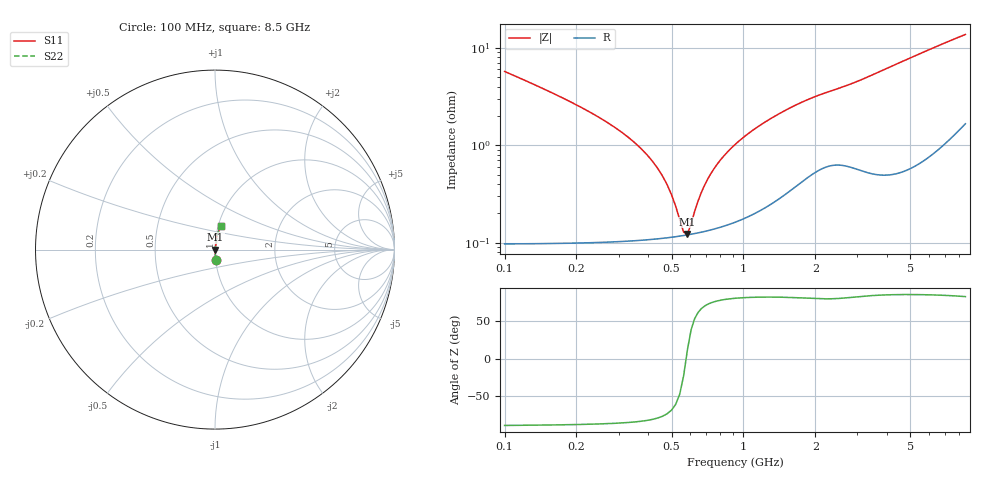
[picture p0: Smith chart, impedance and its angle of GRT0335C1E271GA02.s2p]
!Murata Part Number: GRT0335C1E271GA02
!These Parameters are Measured in Series Mode Connection
!Data Generated on Jun 19, 2026
!  o--ll--o
!Port1  Port2
!  o------o
!Operation Temp=25[degC], DC Bias Voltage=0[V]
!Freq. Start=100[MHz] Stop=9[GHz] 401[Steps]
# Hz S RI R 50
!Freq.(Hz) S11(Real) S11(Imag) S21(Real) S21(Imag) S12(Real) S12(Imag) S22(Real) S22(Imag)
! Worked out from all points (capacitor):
!   401 points, 100 MHz to 8.5 GHz, reference 50 ohm
!   read as one part in series: C = 270 pF near 142 MHz
!   lowest |Z| = 123 mohm at 583 MHz (marker M1)
!   series resonance near 575.7 MHz, so ESL is about 280 pH
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1e8  0.00422 -0.0569  0.9958 0.0569  0.9958 0.0569  0.00422 -0.0569
1.42e8  0.00249 -0.0389  0.9975 0.0389  0.9975 0.0389  0.00249 -0.0389
2.05e8  0.00162 -0.025  0.9984 0.025  0.9984 0.025  0.00162 -0.025
3.94e8  0.00113 -0.00794  0.9989 0.00794  0.9989 0.00794  0.00113 -0.00794
4.57e8  0.00113 -0.00476  0.9989 0.00476  0.9989 0.00476  0.00113 -0.00476
5.41e8  0.00117 -0.00127  0.9988 0.00127  0.9988 0.00127  0.00117 -0.00127
5.62e8  0.00119 -0.000488  0.9988 0.000488  0.9988 0.000488  0.00119 -0.000488
5.83e8  0.0012 0.000263  0.9988 -0.000263  0.9988 -0.000263  0.0012 0.000263
6.04e8  0.00122 0.000987  0.9988 -0.000987  0.9988 -0.000987  0.00122 0.000987
6.67e8  0.00129 0.00303  0.9987 -0.00303  0.9987 -0.00303  0.00129 0.00303
7.3e8  0.00138 0.00491  0.9986 -0.00491  0.9986 -0.00491  0.00138 0.00491
7.93e8  0.00147 0.00667  0.9985 -0.00667  0.9985 -0.00667  0.00147 0.00667
8.77e8  0.00163 0.00888  0.9984 -0.00888  0.9984 -0.00888  0.00163 0.00888
9.82e8  0.00185 0.0115  0.9981 -0.0115  0.9981 -0.0115  0.00185 0.0115
1.129e9  0.00224 0.0148  0.9978 -0.0148  0.9978 -0.0148  0.00224 0.0148
1.507e9  0.00367 0.0226  0.9963 -0.0226  0.9963 -0.0226  0.00367 0.0226
2.032e9  0.00635 0.0313  0.9937 -0.0313  0.9937 -0.0313  0.00635 0.0313
2.914e9  0.00762 0.043  0.9924 -0.043  0.9924 -0.043  0.00762 0.043
4.3e9  0.00939 0.0657  0.9906 -0.0657  0.9906 -0.0657  0.00939 0.0657
5.707e9  0.0149 0.0886  0.9851 -0.0886  0.9851 -0.0886  0.0149 0.0886
7.114e9  0.0231 0.1101  0.9769 -0.1101  0.9769 -0.1101  0.0231 0.1101
8.5e9  0.0336 0.1292  0.9664 -0.1292  0.9664 -0.1292  0.0336 0.1292
